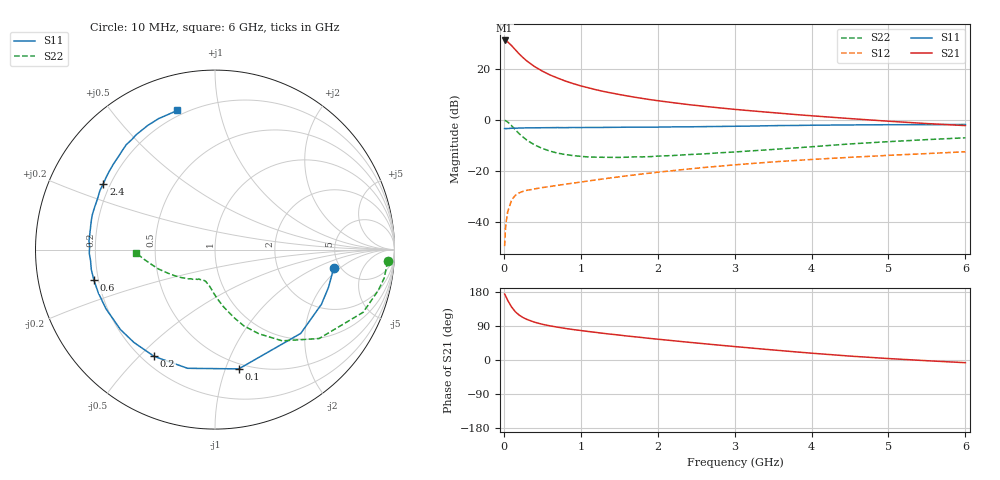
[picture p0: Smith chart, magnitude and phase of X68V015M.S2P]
! SIEMENS Small Signal Semiconductors
! BFP193W
! Si NPN RF Bipolar Junction Transistor in SOT343
! VCE = 8 V  IC = 15 mA
! Common Emitter S-Parameters:  April 1994
# GHz  S  MA  R  50
!  f  S11  S21  S12  S22
! GHz  MAG  ANG  MAG  ANG  MAG  ANG  MAG  ANG
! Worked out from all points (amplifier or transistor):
!   40 points, 10 MHz to 6 GHz, reference 50 ohm
!   highest |S21| = 31.0 dB at 10 MHz (marker M1)
!   |S21| within 3 dB of that: start of sweep to 129.9 MHz
!   unconditionally stable (mu >= 1): 1.171 GHz to 4.435 GHz
!   at 200 MHz: K = 0.28, MSG = 27.2 dB, |S12| = -28.7 dB
!   at 1.5 GHz: K = 1.08, MAG = 14.4 dB, |S12| = -22.4 dB
!   at 6 GHz: K = 0.94, MSG = 5.1 dB, |S12| = -12.6 dB
!   S11 on the Smith chart (normalised r, x): 10 MHz: 4.39, -1.66; 100 MHz: 0.45, -1.11; 200 MHz: 0.25, -0.55; 600 MHz: 0.18, -0.12; 2.4 GHz: 0.17, +0.27; 6 GHz: 0.17, +0.75
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0.01  0.6692 -9.0  35.68 174.1  0.0033 83.9  0.9644 -3.9
0.02  0.6664 -18.5  35.53 170.4  0.0068 80.0  0.9558 -9.6
0.03  0.6667 -27.2  34.98 166.1  0.0098 78.5  0.9372 -14.1
0.05  0.668 -44.3  33.45 157.5  0.0156 70.6  0.8966 -22.9
0.1  0.6777 -78.7  28.32 140.0  0.0263 56.3  0.7629 -40.5
0.15  0.6788 -103.0  23.39 127.2  0.0329 47.5  0.6316 -53.6
0.2  0.6848 -119.7  19.36 118.4  0.0367 42.0  0.5286 -62.5
0.25  0.6867 -131.1  16.43 112.0  0.0392 38.5  0.4552 -69.2
0.3  0.6899 -139.7  14.09 107.1  0.0411 37.0  0.3944 -74.3
0.4  0.6912 -151.5  10.96 99.7  0.0438 35.8  0.3193 -81.9
0.5  0.6934 -159.8  8.945 94.3  0.0465 36.1  0.2724 -87.5
0.6  0.6959 -165.9  7.521 90.1  0.0488 37.1  0.2414 -91.9
0.8  0.6959 -175.0  5.711 83.3  0.0542 40.0  0.2067 -98.3
1.1  0.7035 176.1  4.202 75.2  0.0627 43.6  0.1853 -105.8
1.3  0.7036 170.9  3.562 70.2  0.069 45.6  0.1825 -109.4
1.6  0.7107 164.3  2.923 63.3  0.0792 47.7  0.1832 -114.2
2.2  0.7205 152.9  2.149 50.9  0.1 49.1  0.1977 -123.9
2.4  0.7226 149.4  1.971 46.9  0.1075 49.0  0.2063 -126.7
3.2  0.7466 136.2  1.496 31.9  0.137 46.7  0.2431 -140.0
4.5  0.7867 118.4  1.048 10.3  0.1823 40.2  0.3338 -161.2
5.5  0.7965 109.4  0.837 -1.9  0.2159 34.8  0.4055 -173.1
6  0.8037 105.1  0.764 -7.1  0.2341 32.4  0.4401 -177.7
